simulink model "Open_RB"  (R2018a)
settings: Solver=ode45  StartTime=0.0  StopTime=300  RelTol=1e-3  EnableMultiTasking=on
undefined symbols (not defined in the file or in its folder): Ad, Bd, Cd, Dd, Kpr, Kq

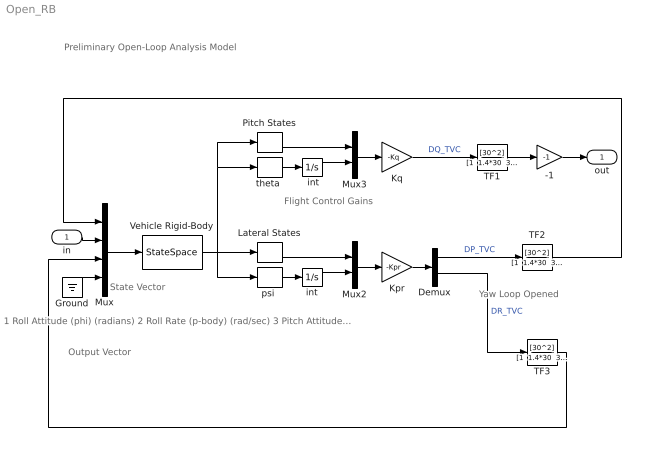
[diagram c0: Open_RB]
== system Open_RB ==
  note: 1 Roll Attitude (phi) (radians) 2 Roll Rate (p-body) (rad/sec) 3 Pitch Attitude (theta) (radians) 4 Pitch Rate (q-body) (rad/sec) 5 Yaw Attitude (psi) (radians) 6 Yaw Rate (r-body) (rad/sec) 7 Angle of attack, alfa, (radians) 8 Angle of sideslip, beta, (radian)
  note: Flight Control Gains
  note: State Vector
  note: Preliminary Open-Loop Analysis Model
  note: Yaw Loop Opened
  note: Output Vector
  in : Inport
  " int" : Integrator
  -1 : Gain  Gain=-1
  Demux : Demux  Outputs=2
  Ground : Ground
  Kpr : Gain  Gain=-Kpr  Multiplication=Matrix(K*u)
  Kq : Gain  Gain=-Kq  Multiplication=Matrix(K*u)
  Lateral States : Selector  InputPortWidth=8  IndexOptions=Index vector (dialog)  Indices="[1  2  5  6  8]"  OutputSizes=1
  Mux : Mux
  Mux2 : Mux  Inputs=[5, 1]
  Mux3 : Mux  Inputs=[3, 1]
  Pitch States : Selector  InputPortWidth=8  IndexOptions=Index vector (dialog)  Indices="[3  4  7]"  OutputSizes=1
  TF1 : TransferFcn  Numerator=[30^2]  Denominator="[1  1.4*30  30^2]"
  TF2 : TransferFcn  Numerator=[30^2]  Denominator="[1  1.4*30  30^2]"
  TF3 : TransferFcn  Numerator=[30^2]  Denominator="[1  1.4*30  30^2]"
  Vehicle Rigid-Body : StateSpace  A=Ad  B=Bd  C=Cd  D=Dd  InitialCondition=0
  int : Integrator
  "psi " : Selector  InputPortWidth=8  IndexOptions=Index vector (dialog)  Indices=[5]  OutputSizes=1
  "theta " : Selector  InputPortWidth=8  IndexOptions=Index vector (dialog)  Indices=[3]  OutputSizes=1
  out : Outport
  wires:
  Mux/1 -> Vehicle Rigid-Body/1
  Vehicle Rigid-Body/1 -> "psi "/1, Lateral States/1, "theta "/1, Pitch States/1
  Kpr/1 -> Demux/1
  Mux2/1 -> Kpr/1
  Lateral States/1 -> Mux2/1
  int/1 -> Mux2/2
  "psi "/1 -> int/1
  Pitch States/1 -> Mux3/1
  "theta "/1 -> " int"/1
  Mux3/1 -> Kq/1
  " int"/1 -> Mux3/2
  Kq/1 -> TF1/1  "DQ_TVC"
  Demux/1 -> TF2/1  "DP_TVC"
  Demux/2 -> TF3/1  "DR_TVC"
  -1/1 -> out/1
  Ground/1 -> Mux/4
  TF2/1 -> Mux/1
  TF1/1 -> -1/1
  in/1 -> Mux/2
  TF3/1 -> Mux/3
